TYPE CHAMBER_IN :
STRUCT
	//C02 	EL1889 16DI
	C02		:ARRAY [1..16] OF BOOL;
	
	
	//C03	EL1889 16DI
	C03		:ARRAY [1..16] OF BOOL;
	
	//C04	EL3318	8TC
	C04		:ARRAY [1..8] OF INT;
	
	
	//C05	EL3318	8TC
	C05		:ARRAY [1..8] OF INT;
	
	
	//C06	EL3164	4AI	0-10V
	C06		:ARRAY [1..4] OF INT;
			
	//C10 	EL9410	POWER MODULE
	
	//C11	EL1918	SPLC+8SDI
	C11		:ARRAY [1..8] OF BOOL;
		
	//C12	EL1904	4SDI
	C12		:ARRAY [1..4] OF BOOL;
	
	
	//C13	EL1904	4SDI
	C13		:ARRAY [1..4] OF BOOL;
	
	//C15	EL3318	8TC
	C15		:ARRAY [1..8] OF INT;
	
END_STRUCT
END_TYPE
